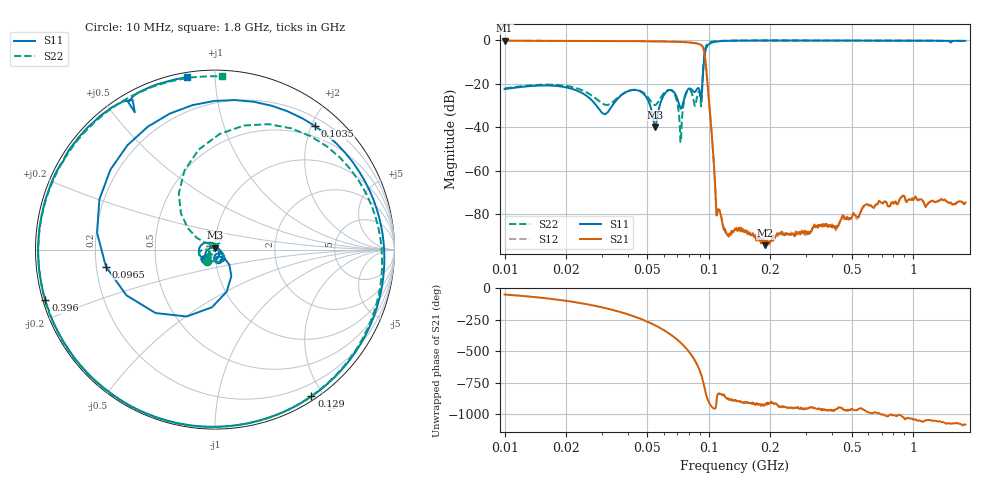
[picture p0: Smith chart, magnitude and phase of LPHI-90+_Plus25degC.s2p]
! Mini-Circuits
! S2P DATA File Format
! Type:LOW PASS FILTER
! Model: LPHI-90+
! All S Parameters are in dB deg format
! TEST CONDITIONS: INPUT POWER = 0 dBm,  +25deg C
# MHz S DB R 50
!Frequency  S11 dB  S11 DEG  S21 dB  S21 DEG  S12 dB  S12 DEG  S22 dB  S22 DEG
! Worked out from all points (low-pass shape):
!   493 points, 10 MHz to 1.8 GHz, reference 50 ohm
!   highest |S21| = -0.18 dB at 10 MHz (marker M1); lowest = -94.4 dB at 189 MHz (marker M2)
!   |S21| within 3 dB of the highest: start of sweep to 93.43 MHz
!   lowest |S11| = -39.9 dB at 54.5 MHz (marker M3), VSWR 1.02, Z = 50.1 + j1.01 ohm
!   |S11| at or under -10 dB: start of sweep to 94.47 MHz
!   |S22| runs from -47.0 to -0.1 dB; largest |S21 - S12| = 0.001
!   S11 on the Smith chart (normalised r, x): 10 MHz: 0.89, -0.10; 96.5 MHz: 0.24, -0.07; 103.5 MHz: 0.32, +2.06; 129 MHz: 0.05, -1.85; 396 MHz: 0.01, -0.15; 1.8 GHz: 0.02, +0.85
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10  -22.45 -134.6  -0.18 -50.0  -0.18 -50.0  -22.15 -125.3
24  -24.32 137.1  -0.27 -120.4  -0.26 -120.4  -23.00 -179.3
38  -24.67 -85.8  -0.34 164.7  -0.33 164.7  -24.59 -122.5
47  -24.00 -150.3  -0.41 112.8  -0.41 112.8  -23.69 -145.5
54.5  -39.87 82.1  -0.46 65.8  -0.46 65.8  -29.82 -119.3
56.5  -32.86 2.6  -0.48 52.5  -0.48 52.5  -28.32 -99.9
67  -23.50 -86.2  -0.64 -23.9  -0.63 -23.9  -24.02 -128.0
73  -31.55 -64.0  -0.75 -74.9  -0.74 -74.9  -46.97 -33.6
82  -22.50 -60.2  -1.08 -169.0  -1.07 -169.0  -23.80 -89.1
88.5  -21.98 -69.3  -1.60 97.2  -1.59 97.2  -24.15 73.3
92.5  -22.67 -43.0  -2.53 12.5  -2.52 12.5  -23.11 145.5
96.5  -4.22 -171.1  -10.95 -114.2  -10.94 -114.2  -2.97 76.8
99.5  -1.95 108.3  -24.94 -179.0  -24.95 -178.9  -1.13 30.5
103.5  -1.05 51.0  -44.69 136.8  -44.69 136.8  -0.61 -2.6
109.5  -0.56 5.3  -80.15 -145.4  -80.40 -144.7  -0.35 -31.5
129  -0.19 -56.7  -87.78 -161.1  -88.00 -168.3  -0.13 -76.7
135  -0.16 -67.0  -87.44 -167.3  -87.00 -173.8  -0.12 -84.9
189  -0.09 -114.5  -94.44 158.2  -94.06 155.5  -0.07 -124.5
320  -0.11 -152.5  -86.50 135.4  -86.92 136.6  -0.10 -157.9
396  -0.12 -163.5  -85.60 114.9  -85.35 110.2  -0.11 -167.9
760  -0.14 166.9  -76.33 69.2  -76.64 71.2  -0.17 162.8
1800  -0.24 99.4  -74.67 -3.2  -74.62 -4.2  -0.30 87.7
